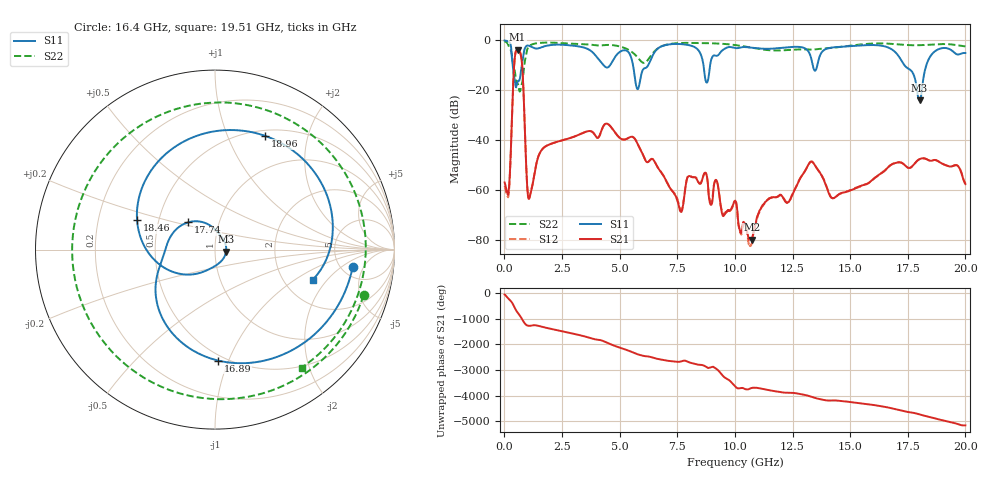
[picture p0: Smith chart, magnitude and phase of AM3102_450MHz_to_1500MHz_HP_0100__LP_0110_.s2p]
!Agilent Technologies,E8364B,MY43040894,A.07.50.67
!Agilent E8364B: A.07.50.67
!Date: Thursday, January 11, 2018 05:36:39
!Correction: S11(Full 2 Port(1,2))
!S21(Full 2 Port(1,2))
!S12(Full 2 Port(1,2))
!S22(Full 2 Port(1,2))
!S2P File: Measurements: S11, S21, S12, S22:
# Hz S  dB  R 50
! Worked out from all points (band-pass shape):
!   1601 points, 10 MHz to 20 GHz, reference 50 ohm
!   highest |S21| = -3.76 dB at 572.2 MHz (marker M1); lowest = -80.0 dB at 10.73 GHz (marker M2)
!   |S21| within 3 dB of the highest: 454.7 MHz to 730.8 MHz (276.2 MHz wide, 46.6 % of centre)
!   lowest |S11| = -24.0 dB at 18.01 GHz (marker M3), VSWR 1.13, Z = 56.6 - j1.3 ohm
!   |S11| at or under -10 dB: 357.1 MHz to 755.8 MHz (398.7 MHz wide, 71.6 % of centre); 5.581 GHz to 6.239 GHz (658.1 MHz wide, 11.1 % of centre); 17.36 GHz to 18.3 GHz (948.2 MHz wide, 5.32 % of centre)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
!   |S22| runs from -20.5 to -0.4 dB; largest |S21 - S12| = 0.0015
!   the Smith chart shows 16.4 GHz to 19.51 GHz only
!   S11 on the Smith chart (normalised r, x): 16.4 GHz: 6.31, -3.06; 16.89 GHz: 0.46, -0.92; 17.74 GHz: 0.71, +0.23; 18.46 GHz: 0.38, +0.16; 18.96 GHz: 0.57, +1.38; 19.51 GHz: 2.88, -1.42
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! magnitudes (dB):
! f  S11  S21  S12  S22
! 10 MHz  -0.1  -57.0  -58.4  -0.4
! 184.9 MHz  -0.6  -60.9  -61.8  -2.3
! 572.2 MHz  -16.6  -3.8  -3.8  -17.5
! 759.6 MHz  -9.8  -8.9  -8.9  -17.4
! 1.084 GHz  -2.2  -63.4  -62.9  -2.3
! 3.346 GHz  -2.7  -37.4  -37.4  -1.5
! 5.782 GHz  -19.6  -41.6  -41.6  -6.9
! 6.682 GHz  -3.1  -51.4  -51.4  -3.1
! 8.781 GHz  -17.0  -54.3  -54.4  -1.1
! 10.01 GHz  -3.1  -64.4  -65.1  -1.9
! 10.73 GHz  -3.0  -80.0  -81.6  -3.0
! 13.34 GHz  -8.4  -48.7  -48.6  -3.8
! 14.25 GHz  -2.9  -63.4  -63.4  -3.0
! 16.4 GHz  -2.2  -53.1  -52.9  -1.3
! 16.68 GHz  -3.0  -50.7  -50.7  -1.3
! 16.89 GHz  -4.2  -49.4  -49.4  -1.5
! 17.74 GHz  -13.5  -50.1  -50.0  -2.0
! 18.01 GHz  -24.0  -47.7  -47.7  -2.0
! 18.46 GHz  -6.7  -48.3  -48.3  -1.8
! 18.96 GHz  -3.2  -49.3  -49.3  -1.5
! 19.51 GHz  -4.9  -50.2  -50.2  -1.8
! 20 GHz  -5.1  -57.7  -57.4  -2.4
